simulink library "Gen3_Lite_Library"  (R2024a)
settings: Solver=VariableStepAuto  StartTime=0.0  StopTime=10.0  RelTol=1e-3
libraries: $bdroot x1

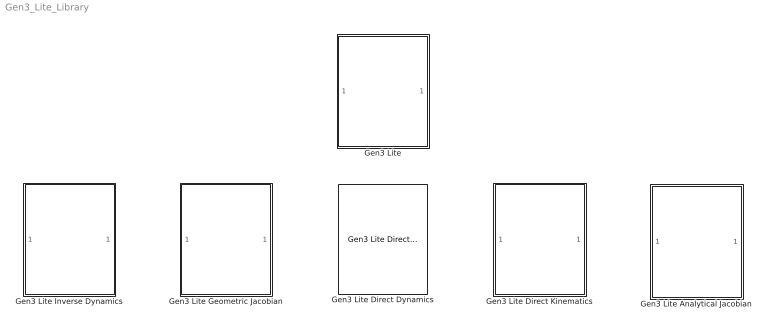
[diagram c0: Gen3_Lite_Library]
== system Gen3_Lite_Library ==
  Gen3 Lite : Subsystem  mask{q0=0, dq0=0}
      mask prompts: q0 "Initial joint position vector"; dq0 "Initial joint velocity vector"
  Gen3 Lite Analytical Jacobian : Subsystem
  Gen3 Lite Direct Dynamics : $bdroot/Gen3 Lite/Gen3 Lite Direct Dynamics
  Gen3 Lite Direct Kinematics : Subsystem
  Gen3 Lite Geometric Jacobian : Subsystem
  Gen3 Lite Inverse Dynamics : Subsystem

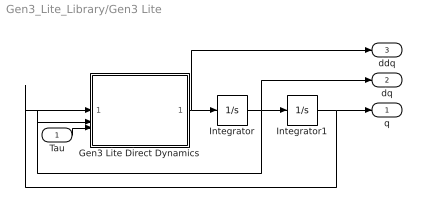
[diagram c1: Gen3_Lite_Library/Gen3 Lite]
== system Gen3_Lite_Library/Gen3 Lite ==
  Tau : Inport
  Gen3 Lite Direct Dynamics : Subsystem
  Integrator : Integrator  InitialCondition=dq0
  Integrator1 : Integrator  InitialCondition=q0
  q : Outport
  dq : Outport  Port=2
  ddq : Outport  Port=3
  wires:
  Integrator1/1 -> q/1, Gen3 Lite Direct Dynamics/1(q)
  Integrator/1 -> dq/1, Gen3 Lite Direct Dynamics/2(dq), Integrator1/1
  Gen3 Lite Direct Dynamics/1(ddq) -> ddq/1, Integrator/1
  Tau/1 -> Gen3 Lite Direct Dynamics/3(Tau)

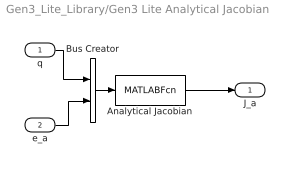
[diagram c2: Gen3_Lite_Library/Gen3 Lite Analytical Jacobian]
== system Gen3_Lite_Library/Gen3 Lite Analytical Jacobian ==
  q : Inport  PortDimensions=[6 1]
  e_a : Inport  Port=2  PortDimensions=[3 1]
  Analytical Jacobian : MATLABFcn  MATLABFcn=Analytical_Jacobian_Gen3_Lite  OutputDimensions=[6 6]  Output1D=off
  Bus Creator : BusCreator  Inputs=2
  J_a : Outport  PortDimensions=[6 6]
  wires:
  Analytical Jacobian/1 -> J_a/1
  Bus Creator/1 -> Analytical Jacobian/1
  q/1 -> Bus Creator/1
  e_a/1 -> Bus Creator/2

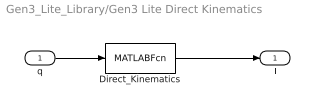
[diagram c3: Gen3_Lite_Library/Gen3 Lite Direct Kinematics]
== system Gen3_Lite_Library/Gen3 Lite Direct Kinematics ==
  q : Inport  PortDimensions=[6 1]
  Direct_Kinematics : MATLABFcn  MATLABFcn=Direct_Kinematics_Gen3_Lite  OutputDimensions=[4 4]  Output1D=off
  T : Outport  PortDimensions=[4 4]
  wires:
  q/1 -> Direct_Kinematics/1
  Direct_Kinematics/1 -> T/1

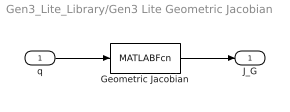
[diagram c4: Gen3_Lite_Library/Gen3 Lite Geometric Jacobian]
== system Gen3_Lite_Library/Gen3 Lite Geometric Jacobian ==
  q : Inport  PortDimensions=[6 1]
  Geometric Jacobian : MATLABFcn  MATLABFcn=Geometric_Jacobian_Gen3_Lite  OutputDimensions=[6 6]  Output1D=off
  J_G : Outport  PortDimensions=[6 6]
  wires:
  Geometric Jacobian/1 -> J_G/1
  q/1 -> Geometric Jacobian/1

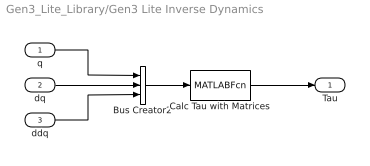
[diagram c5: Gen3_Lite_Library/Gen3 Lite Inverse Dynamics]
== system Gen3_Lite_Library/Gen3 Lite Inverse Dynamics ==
  q : Inport  PortDimensions=[6 1]
  dq : Inport  Port=2  PortDimensions=[6 1]
  ddq : Inport  Port=3  PortDimensions=[6 1]
  Bus Creator2 : BusCreator  Inputs=3
  Calc Tau with Matrices : MATLABFcn  MATLABFcn=Inverse_Dyn_with_Matrices_Gen3_Lite  OutputDimensions=[6 1]  Output1D=off
  Tau : Outport  PortDimensions=[6 1]
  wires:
  dq/1 -> Bus Creator2/2
  Bus Creator2/1 -> Calc Tau with Matrices/1
  ddq/1 -> Bus Creator2/3
  q/1 -> Bus Creator2/1
  Calc Tau with Matrices/1 -> Tau/1

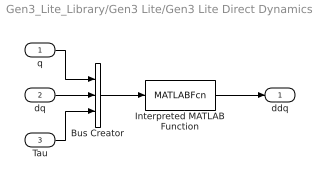
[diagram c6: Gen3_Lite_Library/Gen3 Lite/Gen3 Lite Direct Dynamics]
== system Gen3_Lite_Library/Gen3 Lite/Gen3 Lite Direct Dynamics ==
  q : Inport
  dq : Inport  Port=2
  Tau : Inport  Port=3
  Bus Creator : BusCreator  Inputs=3
  Interpreted MATLAB Function : MATLABFcn  MATLABFcn=direct_gen3_lite_dynamics  OutputDimensions=6
  ddq : Outport
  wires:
  dq/1 -> Bus Creator/2
  Tau/1 -> Bus Creator/3
  Interpreted MATLAB Function/1 -> ddq/1
  Bus Creator/1 -> Interpreted MATLAB Function/1
  q/1 -> Bus Creator/1
